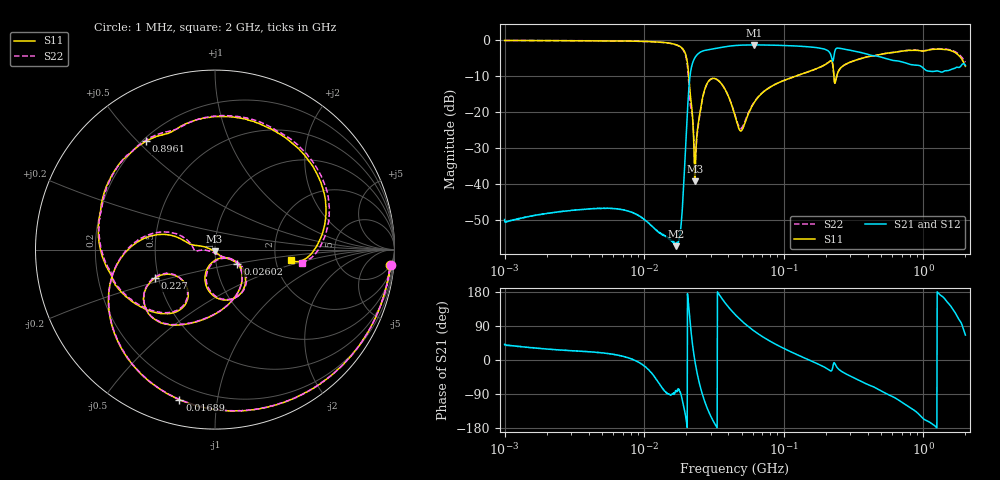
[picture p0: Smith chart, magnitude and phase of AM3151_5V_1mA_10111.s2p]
! Date/Time: Fri Jun 26 10:58:38 2020
! Network Analyzer:  Rev:
! Sweep from 1000000.0 to 2000000000.0, 1601 Points ! Power Supply: 0 V, 0 A
# HZ S DB R 50
!freq MagS11 AngS11 MagS21 AngS21 MagS12 AngS12 MagS22 AngS22
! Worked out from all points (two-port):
!   1601 points, 1 MHz to 2 GHz, reference 50 ohm
!   highest |S21| = -1.38 dB at 61.19 MHz (marker M1); lowest = -57.4 dB at 16.81 MHz (marker M2)
!   |S21| within 3 dB of the highest: 23.61 MHz to 218.1 MHz (194.5 MHz wide, 161 % of centre); 229.1 MHz to 437.8 MHz (208.7 MHz wide, 62.6 % of centre)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
!   lowest |S11| = -39.4 dB at 23.11 MHz (marker M3), VSWR 1.02, Z = 49.7 - j1.04 ohm
!   |S11| at or under -10 dB: 20.85 MHz to 123.5 MHz (102.7 MHz wide, 142 % of centre); 228.6 MHz to 239.5 MHz (10.93 MHz wide, 4.67 % of centre)
!   |S22| runs from -34.6 to -0.2 dB; largest |S21 - S12| = 0.0091
!   S11 on the Smith chart (normalised r, x): 1 MHz: 5, -22; 16.89 MHz: 0.12, -0.78; 26.02 MHz: 1.27, -0.20; 227 MHz: 0.48, -0.17; 896.1 MHz: 0.21, +0.53; 2 GHz: 2.44, -0.34
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1000000  -0.17 -4.9  -49.99 41.3  -50.61 39.7  -0.16 -4.9
3555161  -0.23 -16.6  -47.21 23.2  -47.17 22.8  -0.22 -16.6
1.263916e7  -0.59 -65.6  -53.48 -58.9  -53.40 -59.3  -0.60 -65.7
1.680764e7  -1.29 -102.4  -57.40 -81.7  -57.56 -84.4  -1.33 -103.3
1.688767e7  -1.32 -103.4  -56.64 -80.7  -57.02 -84.8  -1.36 -104.3
1.830811e7  -2.00 -124.1  -52.20 -91.1  -52.21 -91.1  -2.09 -125.9
2.003748e7  -4.72 -167.3  -25.80 -160.5  -25.78 -160.5  -5.19 -172.0
2.18263e7  -18.20 168.2  -7.55 63.2  -7.54 63.2  -19.39 -175.8
2.310668e7  -39.39 -104.0  -4.92 -3.8  -4.92 -3.9  -34.61 -120.8
2.602052e7  -16.64 -31.8  -3.16 -88.6  -3.15 -88.6  -16.85 -29.4
3.237582e7  -10.81 -77.4  -2.39 -171.2  -2.39 -171.3  -10.83 -75.5
4.493426e7  -21.43 -107.7  -1.56 119.5  -1.56 119.5  -21.16 -104.2
4.988463e7  -25.22 -62.1  -1.46 103.2  -1.46 103.2  -24.57 -61.4
6.11902e7  -17.50 -30.5  -1.38 76.7  -1.41 76.7  -17.39 -31.1
1.589914e8  -8.49 -94.6  -2.02 -3.3  -2.00 -3.4  -8.51 -94.9
2.270438e8  -8.68 -154.8  -5.37 -10.1  -5.35 -10.2  -8.53 -155.4
3.211579e8  -5.75 -141.0  -3.13 -47.9  -3.14 -48.1  -5.78 -141.9
5.652395e8  -3.64 170.9  -5.43 -92.1  -5.40 -92.0  -3.63 169.0
8.961029e8  -2.90 122.5  -7.03 -137.7  -7.02 -137.9  -2.85 120.1
1.329226e9  -2.58 70.1  -8.91 170.6  -8.86 170.4  -2.47 67.8
1.661753e9  -3.34 26.1  -7.96 128.9  -7.84 128.0  -3.13 25.9
2e9  -7.36 -7.6  -7.08 65.7  -7.19 65.6  -6.21 -8.7
